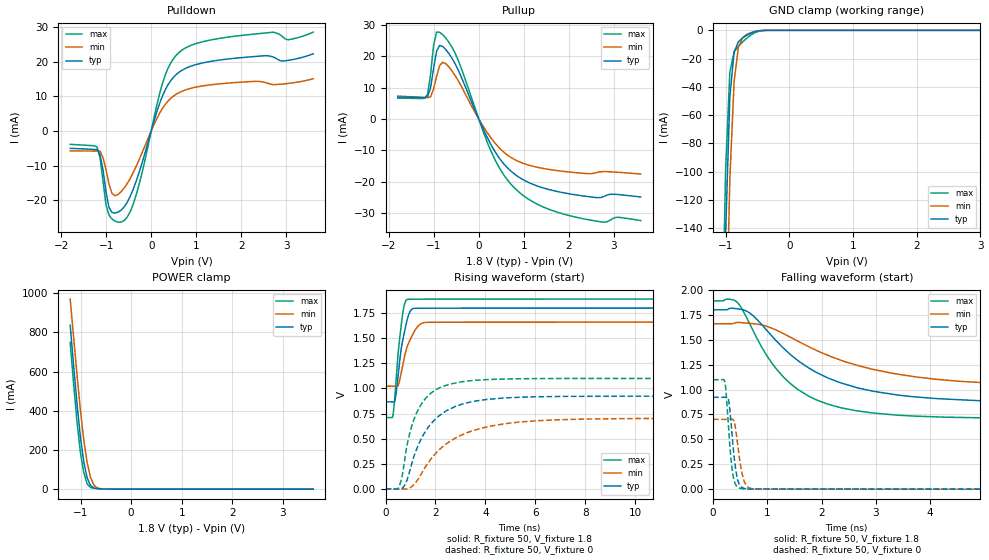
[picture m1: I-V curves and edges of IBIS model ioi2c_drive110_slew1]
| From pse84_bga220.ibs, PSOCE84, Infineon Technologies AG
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[Model] ioi2c_drive110_slew1
Model_type I/O
Enable   Active-High
Vinl  =  0.54
Vinh  =  1.26
Vmeas =  0.9
Cref  =  15e-12
| Capacitance   typ   min   max
C_comp   8.55364e-13 8.30808e-13 8.84570e-13
| Variables   typ   min   max
[GND Clamp Reference]   0   0   0
[POWER Clamp Reference]   1.8   1.66   1.89
[Pulldown Reference]   0   0   0
[Pullup Reference]   1.8   1.66   1.89
[Temperature Range]   25   125   -40
[Voltage Range]   1.8   1.66   1.89
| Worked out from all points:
|   slope of the pulldown table from 0 to 0.27 V, typ, clamps not added: 25.3 ohm
|   slope of the pullup table from 0 to 0.27 V, typ, clamps not added: 33.2 ohm
|   GND clamp passes 1 mA (typ) near -0.55 V on its own axis
|   POWER clamp passes 1 mA (typ) near -0.55 V on its own axis
|   falling waveform, R_fixture 50, V_fixture 1.8: 20-80 % time 1.48ns typ, 2.05ns min, 1.05ns max; typ from 1.8 V to 0.867 V
|   falling waveform, R_fixture 50, V_fixture 0: 20-80 % time 100ps typ, 115ps min, 93ps max; typ from 0.922 V to 0 V
|   rising waveform, R_fixture 50, V_fixture 1.8: 20-80 % time 327ps typ, 453ps min, 256ps max; typ from 0.867 V to 1.8 V
|   rising waveform, R_fixture 50, V_fixture 0: 20-80 % time 1.22ns typ, 1.87ns min, 808ps max; typ from 0 V to 0.922 V
[GND Clamp]
| Voltage   I(typ)   I(min)   I(max)
-1.204V   -750.5mA   -844.3mA   -692.2mA
-1.07V    -311.8mA   -416.8mA   -250.3mA
-1.003V   -144.6mA   -236.7mA   -99.35mA
-936.6mV  -47.15mA   -105.3mA   -29.57mA
-869.7mV  -15.32mA   -36.11mA   -15.4mA
-802.8mV  -8.178mA   -12.13mA   -11.32mA
-735.9mV  -5.345mA   -5.294mA   -8.218mA
-669mV    -3.361mA   -2.852mA   -5.471mA
-535.2mV  -838.5uA   -772.4uA   -1.486mA
-401.4mV  -47.36uA   -84.85uA   -76.78uA
3.6V      0A         0A         0A
[POWER Clamp]
| Voltage   I(typ)   I(min)   I(max)
-1.204V   837.3mA    970.7mA    749.2mA
-1.137V   634.9mA    778.2mA    540.5mA
-1.07V    440.1mA    587.4mA    346.5mA
-1.003V   270mA      407mA      190.9mA
-936.6mV  141.8mA    252.7mA    85.92mA
-869.7mV  58.74mA    136.5mA    26.66mA
-802.8mV  18.35mA    60.36mA    8.197mA
-735.9mV  5.885mA    21mA       4.755mA
-669mV    2.866mA    6.628mA    3.138mA
-334.5mV  12.31uA    45.7uA     5.857uA
3.6V      0A         0A         0A
[Pulldown]
| Voltage   I(typ)   I(min)   I(max)
-1.8V     -5.031mA   -5.777mA   -3.872mA
-1.204V   -5.388mA   -5.825mA   -4.584mA
-1.07V    -11.24mA   -7.714mA   -14.52mA
-1.003V   -17.74mA   -11.24mA   -21.49mA
-936.6mV  -22.2mA    -15.46mA   -24.36mA
-802.8mV  -23.75mA   -18.74mA   -26.09mA
-669mV    -22.92mA   -17.59mA   -26.38mA
-401.4mV  -16.91mA   -12.1mA    -21.21mA
248.3mV   10.03mA    6.478mA    13.65mA
558.6mV   16.35mA    10.65mA    21.94mA
1.49V     20.45mA    13.59mA    26.71mA
3.6V      22.33mA    15.11mA    28.6mA
[Pullup]
| Voltage   I(typ)   I(min)   I(max)
-1.8V     7.005mA    7.261mA    6.626mA
-1.137V   7.083mA    6.76mA     7.811mA
-1.07V    9.886mA    7.034mA    14.08mA
-1.003V   15.99mA    9.505mA    23.38mA
-936.6mV  21.53mA    13.57mA    27.68mA
-869.7mV  23.43mA    16.94mA    27.64mA
-735.9mV  22.16mA    17.65mA    25.83mA
-468.3mV  15.98mA    12.5mA     19.13mA
310.3mV   -9.196mA   -6.788mA   -11.49mA
806.9mV   -17.72mA   -13.02mA   -22.19mA
1.996V    -23.84mA   -16.9mA    -30.76mA
3.6V      -24.91mA   -17.59mA   -32.41mA
[Ramp]
dV/dt_r   0.553161/1.22219n  0.420206/1.86832n  0.659218/0.80818n
dV/dt_f   0.559864/1.47777n  0.382426/2.05457n  0.708163/1.04552n
R_load = 50
[Falling Waveform]
R_fixture = 50
V_fixture = 1.8
V_fixture_min = 1.66
V_fixture_max = 1.89
| Time   V(typ)   V(min)   V(max)
0s        1.8V       1.66V      1.89V
434ps     1.812V     1.673V     1.881V
745.2ps   1.738V     1.661V     1.583V
1.17ns    1.486V     1.596V     1.204V
1.558ns   1.294V     1.487V     1.002V
2.096ns   1.122V     1.348V     856.7mV
2.673ns   1.016V     1.241V     784.7mV
3.722ns   926.7mV    1.128V     733.3mV
6.441ns   872.8mV    1.039V     709.9mV
800ns     866.9mV    1.023V     709.7mV
[Falling Waveform]
R_fixture = 50
V_fixture = 0
V_fixture_min = 0
V_fixture_max = 0
| Time   V(typ)   V(min)   V(max)
0s        921.9mV    700.3mV    1.099V
217.7ps   921.7mV    700.3mV    1.075V
243.5ps   922.4mV    700.3mV    952.9mV
294.6ps   867.9mV    700.2mV    542.8mV
350ps     545.3mV    701.6mV    203mV
410.7ps   223.5mV    622.2mV    51.68mV
512.4ps   26.39mV    218.6mV    6.613mV
597.9ps   5.254mV    49.68mV    2.326mV
978.2ps   1.2mV      1.183mV    782.2uV
800ns     6.766nV    466.7nV    2.504nV
[Rising Waveform]
R_fixture = 50
V_fixture = 1.8
V_fixture_min = 1.66
V_fixture_max = 1.89
| Time   V(typ)   V(min)   V(max)
0s        866.9mV    1.023V     709.7mV
301.5ps   867.1mV    1.023V     738.7mV
396.6ps   904.4mV    1.023V     988.6mV
530.1ps   1.188V     1.046V     1.415V
629.2ps   1.397V     1.158V     1.632V
758.2ps   1.564V     1.315V     1.838V
826.7ps   1.643V     1.383V     1.88V
988.9ps   1.77V      1.487V     1.888V
1.425ns   1.799V     1.645V     1.889V
800ns     1.8V       1.66V      1.89V
[Rising Waveform]
R_fixture = 50
V_fixture = 0
V_fixture_min = 0
V_fixture_max = 0
| Time   V(typ)   V(min)   V(max)
0s        6.767nV    466.5nV    2.506nV
543.8ps   -2.913mV   -1.403mV   25.44mV
651ps     1.967mV    -2.028mV   111.2mV
799.1ps   51.7mV     -2.128mV   344.2mV
1.037ns   239.7mV    18.9mV     614.1mV
1.614ns   577.3mV    224.9mV    904.8mV
2.442ns   778.2mV    449.2mV    1.032V
3.391ns   864mV      570.5mV    1.077V
7.933ns   921.5mV    694.7mV    1.099V
50ns      921.9mV    700.3mV    1.099V
